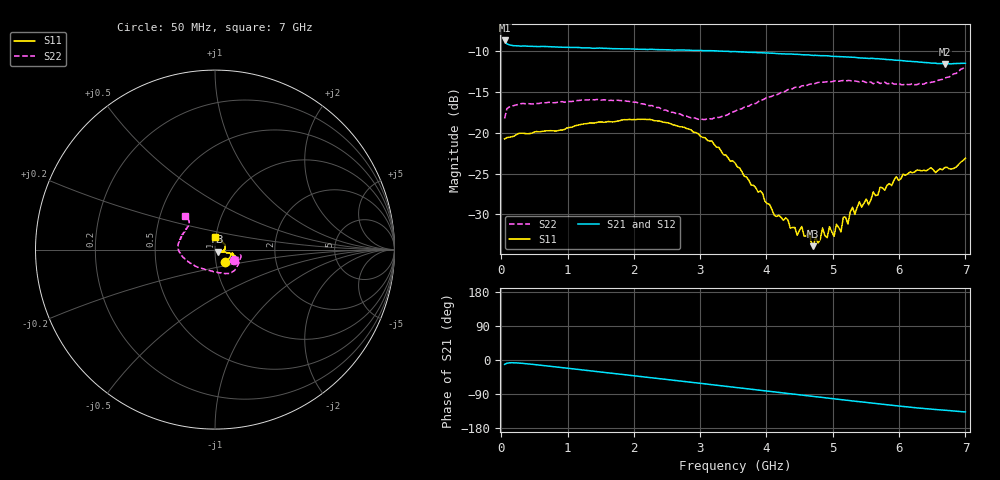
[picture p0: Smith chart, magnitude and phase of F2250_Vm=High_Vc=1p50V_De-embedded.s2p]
! Integrated Device Technology
! Corporate Headquarters
! 6024 Silver Creek Valley Road
! San Jose, CA 95138  USA
! Phone:  1-408-284-8200
! Toll Free:  1-800-223-1366
! Webpage:  http://www.idt.com/
! Timing and RF Division
! 515 Groton Road, Suite 102
! Westford, MA 01886-6024
! Device:  F2250
! Description: Voltage Variable RF Attenuator
! Frequency:  50.0 -  6000.00 MHz
! Package:  3x3 mm Thin QFN Plastic Package: 16 pin
! Ports:  2 RF, 3 DC
!  Pin  1  = GND
!  Pin  2  = NC
!  Pin  3  = RF1  = Port 1
!  Pin  4  = NC
!  Pin  5  = GND
!  Pin  6  = GND
!  Pin  7  = GND
!  Pin  8  = GND
!  Pin  9  = NC
!  Pin 10  = RF2  = Port 2
!  Pin 11  = NC
!  Pin 12  = GND
!  Pin 13  = GND
!  Pin 14  = VCNTRL
!  Pin 15  = VDD
!  Pin 16  = VMODE
! Vcntrl:  1.500 Volts
! Vmode:  +3.300 Volts
! Vdd:  +3.30  Volts
! Current:  1.328 mA
! Data:  The device was measured on a the F2250 evaluation board which has
!  individual transmission lines to the RF pins.  Data was collected
!  using a calibrated network analyzer.  The evaluation board was
!  de-embedded using a TRL calibration technique.
!  The reference plane is the edge of the package pin.
! Misc:  SN 10
!  Action Tracker AT0258
! Date Measured:  2014-11-26
! Date:  2015-10-15  MJV
! Note:
!  Integrated Device Technology supplies this data as a sample of measured
!  data at the package pin for this product.  Your particular data for this
!  product may vary.
!  Data was taken at 25 degrees C.
!  Integrated Device Technology reserves the right to change this data at anytime.
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# GHz S dB R 50
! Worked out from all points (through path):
!   201 points, 50 MHz to 7 GHz, reference 50 ohm
!   highest |S21| = -8.75 dB at 50 MHz (marker M1); lowest = -11.6 dB at 6.687 GHz (marker M2)
!   group delay of S21, straight-line fit = 54.7 ps
!   lowest |S11| = -33.9 dB at 4.707 GHz (marker M3), VSWR 1.04, Z = 51.7 - j1.18 ohm
!   |S11| at or under -10 dB: start of sweep to end of sweep
!   |S22| runs from -18.4 to -12.0 dB; largest |S21 - S12| = 0.0018
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0.05  -20.77 -51.5  -8.75 -11.6  -8.74 -11.6  -18.27 -29.5
0.29325  -20.08 -11.6  -9.44 -8.5  -9.42 -8.5  -16.47 -14.3
1.2315  -18.96 -21.2  -9.66 -26.3  -9.65 -26.3  -16.00 -42.2
2.37825  -18.58 -18.2  -9.87 -48.8  -9.86 -48.9  -16.93 -70.2
2.969  -20.12 -13.4  -9.98 -60.8  -9.98 -60.9  -18.38 -97.9
3.525  -23.70 -14.1  -10.10 -72.3  -10.12 -72.3  -17.39 -132.4
4.11575  -30.07 -22.4  -10.32 -84.3  -10.33 -84.4  -15.42 -159.2
4.46325  -32.53 -30.9  -10.45 -91.3  -10.45 -91.4  -14.46 -169.6
4.637  -31.90 -31.0  -10.51 -94.9  -10.53 -94.9  -14.13 -174.9
4.7065  -33.87 -34.2  -10.57 -96.2  -10.54 -96.3  -14.07 -175.9
4.8455  -31.65 -36.1  -10.60 -99.0  -10.60 -99.0  -13.85 -178.9
4.915  -32.83 -38.4  -10.62 -100.5  -10.63 -100.4  -13.78 179.1
4.94975  -31.49 -34.3  -10.65 -101.1  -10.65 -101.1  -13.78 178.4
5.1235  -32.13 -32.8  -10.73 -104.6  -10.71 -104.7  -13.67 174.1
5.15825  -30.32 -32.9  -10.74 -105.2  -10.71 -105.4  -13.64 173.7
5.22775  -31.18 -26.8  -10.76 -106.7  -10.76 -106.7  -13.64 171.9
5.29725  -29.12 -21.1  -10.79 -108.0  -10.77 -108.1  -13.73 170.4
5.332  -29.98 -20.0  -10.81 -108.7  -10.81 -108.8  -13.70 169.4
5.4015  -28.45 -16.3  -10.88 -110.0  -10.84 -110.1  -13.82 167.2
5.85325  -26.23 -5.2  -11.09 -118.7  -11.09 -118.8  -14.01 155.1
6.68725  -24.26 47.4  -11.61 -132.5  -11.60 -132.6  -13.35 132.0
7  -23.13 88.6  -11.53 -137.1  -11.54 -137.3  -11.96 131.8
